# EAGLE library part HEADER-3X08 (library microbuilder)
3x8 0.1" Headers Male - 4UCON: 01058
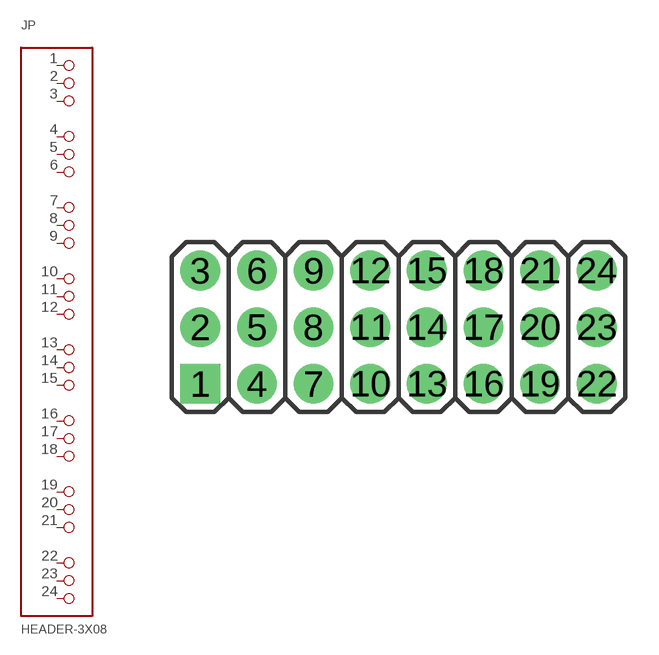
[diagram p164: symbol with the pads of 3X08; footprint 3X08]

Designator prefix JP

## HEADER-3X08  [3X08]
1  1  pas
2  2  pas
3  3  pas
4  4  pas
5  5  pas
6  6  pas
7  7  pas
8  8  pas
9  9  pas
10  10  pas
11  11  pas
12  12  pas
13  13  pas
14  14  pas
15  15  pas
16  16  pas
17  17  pas
18  18  pas
19  19  pas
20  20  pas
21  21  pas
22  22  pas
23  23  pas
24  24  pas

## Footprint 3X08 (pad centres in mm)
drill 1 pad 1.778 square: 1 -8.89,-2.54
drill 1 pad 1.778: 2 -8.89,0; 3 -8.89,2.54; 4 -6.35,-2.54; 5 -6.35,0; 6 -6.35,2.54; 7 -3.81,-2.54; 8 -3.81,0; 9 -3.81,2.54; 10 -1.27,-2.54; 11 -1.27,0; 12 -1.27,2.54; 13 1.27,-2.54; 14 1.27,0; 15 1.27,2.54; 16 3.81,-2.54; 17 3.81,0; 18 3.81,2.54; 19 6.35,-2.54; 20 6.35,0; 21 6.35,2.54; 22 8.89,-2.54; 23 8.89,0; 24 8.89,2.54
